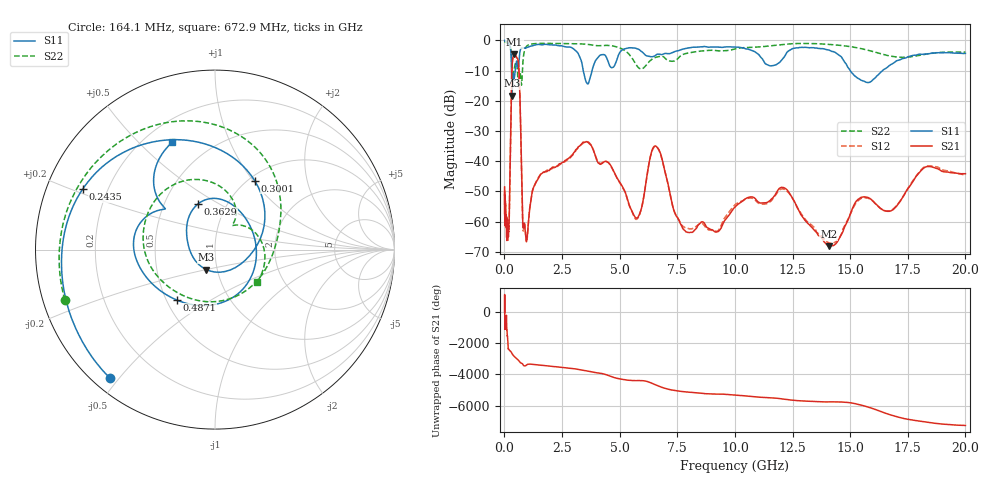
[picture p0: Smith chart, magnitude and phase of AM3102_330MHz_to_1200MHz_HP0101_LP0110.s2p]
! Date/Time: Tue, Sep 11, 2018 5:14 PM
! Network Analyzer: Agilent Technologies E8362B Rev: A.07.50.63
! Sweep from 0.010 to 20.000 GHz, 1601 Points, Sweep Type: LOG
! Power Supply: 4.949 V, 0.001 A
# Hz S DB R 50
!freq MagS11 AngS11 MagS21 AngS21 MagS12 AngS12 MagS22 AngS22
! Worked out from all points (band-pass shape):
!   1601 points, 10 MHz to 20 GHz, reference 50 ohm
!   highest |S21| = -4.64 dB at 430.5 MHz (marker M1); lowest = -68.1 dB at 14.07 GHz (marker M2)
!   |S21| within 3 dB of the highest: 340.1 MHz to 612 MHz (271.9 MHz wide, 57.1 % of centre)
!   lowest |S11| = -18.3 dB at 331.5 MHz (marker M3), VSWR 1.28, Z = 44.2 - j9.96 ohm
!   |S11| at or under -10 dB: 309.4 MHz to 471.2 MHz (161.9 MHz wide, 41.5 % of centre); 3.422 GHz to 3.802 GHz (379.6 MHz wide, 10.5 % of centre); 15.01 GHz to 16.41 GHz (1.4 GHz wide, 8.91 % of centre)
!   |S22| runs from -15.6 to -0.2 dB; largest |S21 - S12| = 0.0098
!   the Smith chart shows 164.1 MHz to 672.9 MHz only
!   S11 on the Smith chart (normalised r, x): 164.1 MHz: 0.05, -0.47; 243.5 MHz: 0.11, +0.22; 300.1 MHz: 1.07, +1.02; 362.9 MHz: 0.73, +0.41; 487.1 MHz: 0.56, -0.36; 672.9 MHz: 0.31, +0.63
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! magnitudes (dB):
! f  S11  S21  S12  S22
! 10 MHz  0.0  -48.5  -50.1  -0.2
! 35.55 MHz  0.0  -58.6  -59.6  -0.4
! 126.4 MHz  -0.4  -61.6  -62.5  -0.9
! 164.1 MHz  -0.7  -63.3  -65.0  -1.1
! 243.5 MHz  -1.8  -44.0  -44.1  -1.8
! 300.1 MHz  -7.1  -17.9  -18.0  -4.0
! 331.5 MHz  -18.3  -8.8  -8.9  -8.0
! 362.9 MHz  -11.3  -6.0  -6.1  -10.7
! 430.5 MHz  -12.4  -4.6  -4.7  -9.1
! 447.2 MHz  -11.4  -4.7  -4.7  -8.4
! 487.1 MHz  -9.1  -4.9  -5.1  -7.5
! 672.9 MHz  -3.8  -18.4  -18.4  -10.6
! 817.6 MHz  -2.5  -62.1  -63.1  -6.0
! 1.59 GHz  -1.4  -44.2  -44.2  -1.0
! 3.617 GHz  -14.4  -33.7  -33.5  -1.3
! 5.652 GHz  -2.5  -58.3  -58.8  -7.2
! 6.58 GHz  -4.8  -35.1  -35.2  -5.6
! 7.882 GHz  -2.6  -63.4  -62.1  -4.3
! 12.09 GHz  -5.9  -48.7  -49.1  -1.3
! 14.07 GHz  -3.2  -68.1  -67.0  -1.3
! 15.7 GHz  -13.9  -51.9  -52.2  -3.1
! 20 GHz  -4.3  -44.1  -44.6  -3.9
